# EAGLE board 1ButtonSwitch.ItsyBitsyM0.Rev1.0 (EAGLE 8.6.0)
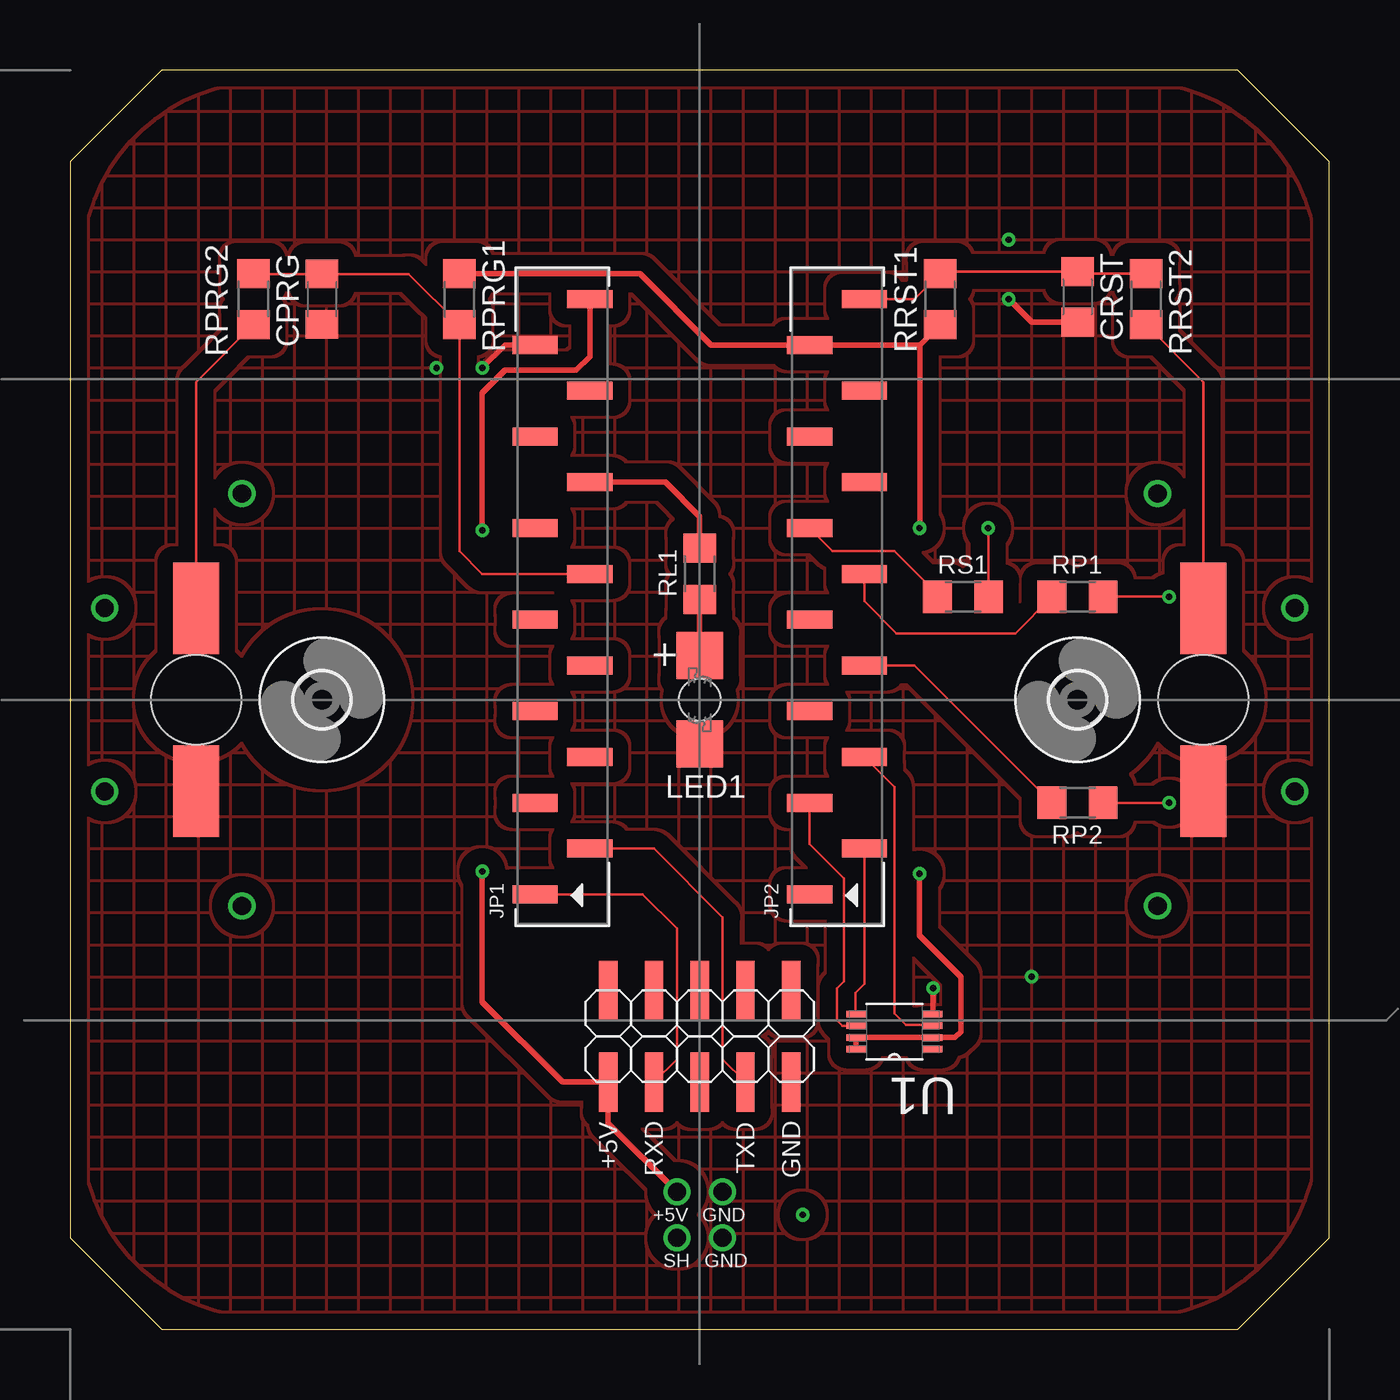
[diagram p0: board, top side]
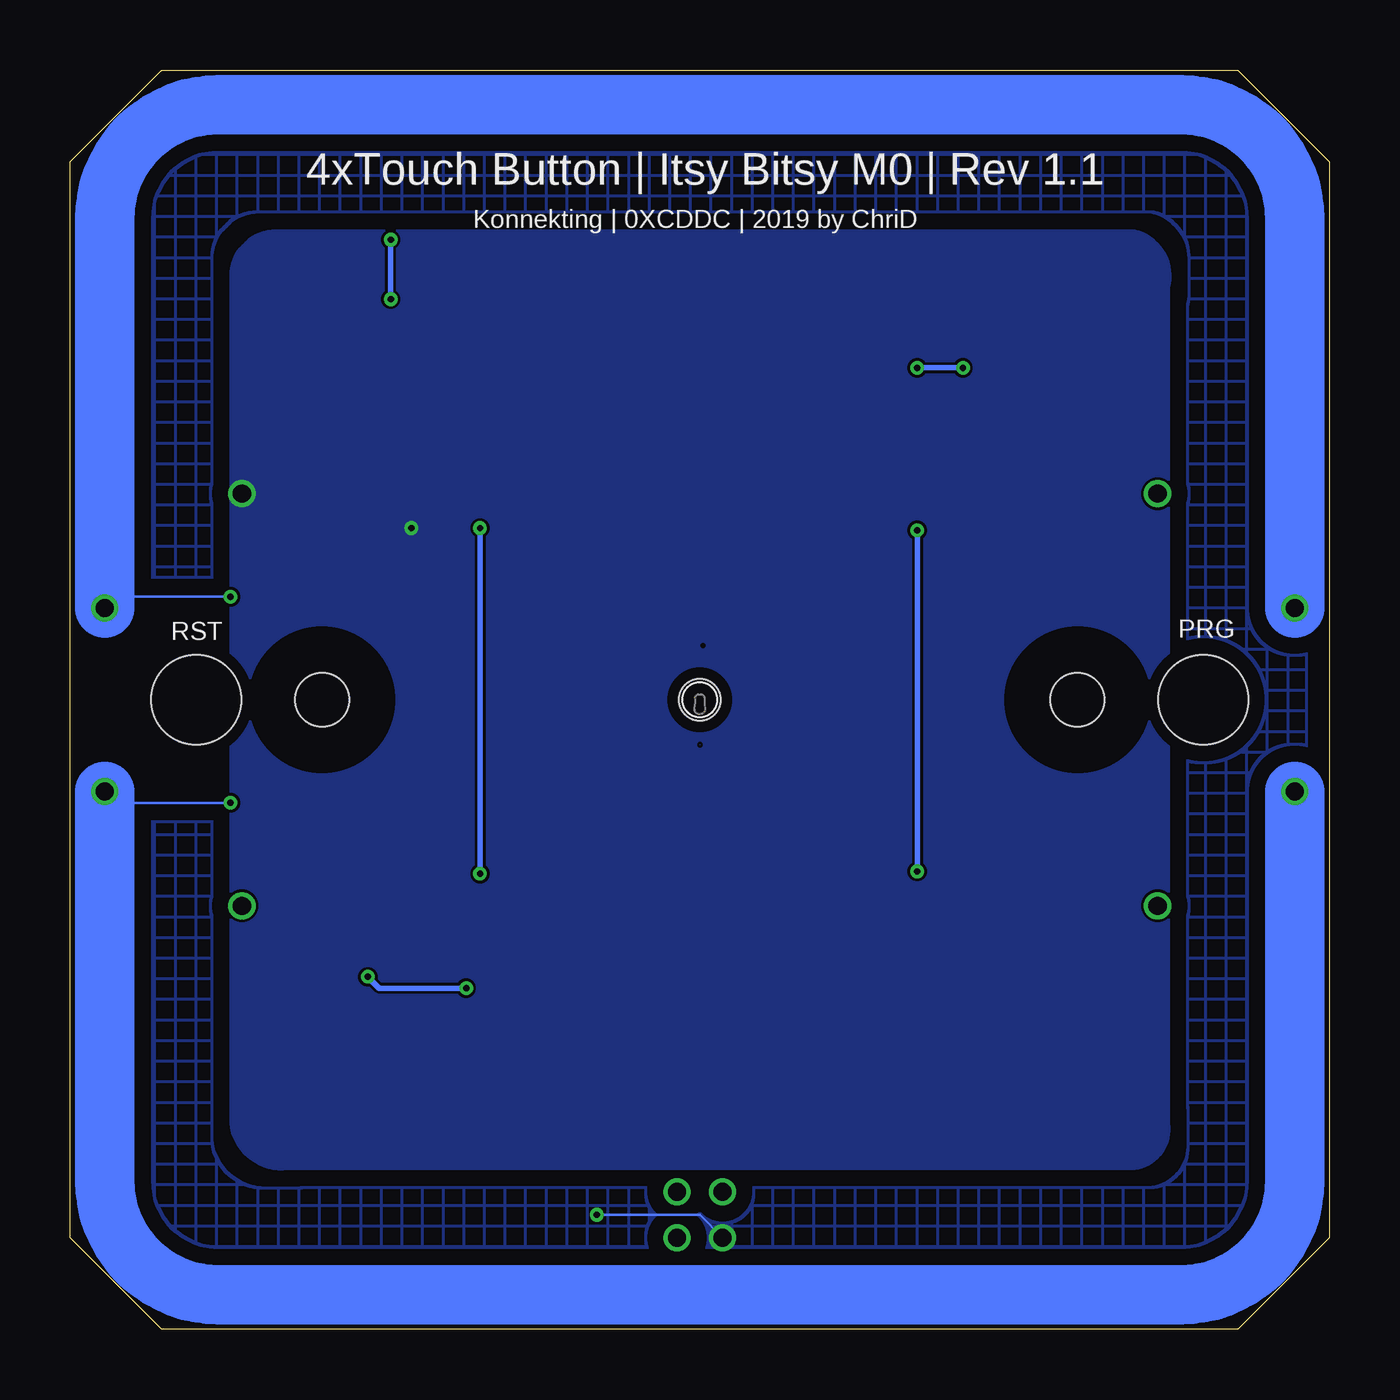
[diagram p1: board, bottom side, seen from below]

Size 69.85 x 69.85 mm. Coordinates in mm from the lower left corner, seen from the top.
Outline: 5.08,69.85 64.77,69.85 69.85,64.77 69.85,5.08 64.77,0 5.08,0 0,5.08 0,64.77 5.08,69.85
Outline: 6.34,69.84 5.08,69.85
Copper layers (1*16): Top 0.035mm / dielectric 1.5mm / Bottom 0.035mm
Design rules "konnektduino": minimum track width 6mil, minimum drill 0.35mm, track to track 6mil, track to pad 6mil, pad to pad 6mil, via to via 6mil, smd to smd 6mil, copper to edge 25mil, drill to drill 6mil, minimum pad ring 10mil, minimum via ring 8mil, stop-mask expansion 1mil, vias tented up to drill 25mil, thermal gap 10mil
Holes 5 mm at 62.87,34.92 6.99,34.92

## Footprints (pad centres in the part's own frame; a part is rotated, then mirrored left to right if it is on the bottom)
C1206 = smd 1.6 x 1.8: 1 -1.4,0; 2 1.4,0
SMD2,54-5,08 = smd 2.54 x 5.08: 1 0,0
1X14_SMT = smd 1 x 2.5: 1 -16.51,1.52; 2 -13.97,-1.52; 3 -11.43,1.52; 4 -8.89,-1.52; 5 -6.35,1.52; 6 -3.81,-1.52; 7 -1.27,1.52; 8 1.27,-1.52; 9 3.81,1.52; 10 6.35,-1.52; 11 8.89,1.52; 12 11.43,-1.52; 13 13.97,1.52; 14 16.51,-1.52
P47F-BOTTOM = smd 2.6 x 2.6: A -2.45,0; C 2.45,0 | hole 2.3: 0,0
R1206 = smd 1.6 x 1.803: 1 -1.422,0; 2 1.422,0
2X05SMD = smd 1.016 x 3.302: 1 -1.27,-3.81; 2 -1.27,1.27; 3 1.27,-3.81; 4 1.27,1.27; 5 3.81,-3.81; 6 3.81,1.27; 7 6.35,-3.81; 8 6.35,1.27; 9 8.89,-3.81; 10 8.89,1.27
SOP65P490X110-8N = smd 1.067 x 0.356: 1 -2.134,0.965; 2 -2.134,0.33; 3 -2.134,-0.33; 4 -2.134,-0.965; 5 2.134,-0.965; 6 2.134,-0.33; 7 2.134,0.33; 8 2.134,0.965
3,0 = hole 3: 0,0

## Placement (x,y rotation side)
CPRG  100nF  [C1206]  13.97,57.15 270 top
CRST  100nF  [C1206]  55.88,57.28 270 top
GND_NRST  0  [SMD2,54-5,08]  6.99,29.84 0 top
GND_PRG  0  [SMD2,54-5,08]  62.87,29.84 0 top
JP1  [1X14_SMT]  27.3,40.64 90 top
JP2  [1X14_SMT]  42.55,40.64 90 top
LED1  LWP4-BOTTOM  [P47F-BOTTOM]  34.92,34.92 270 top
PAD_NRST  0  [SMD2,54-5,08]  62.87,40.01 0 top
PAD_PRG  0  [SMD2,54-5,08]  6.99,40.01 0 top
RL1  330E  [R1206]  34.92,41.91 270 top
RP1  1k  [R1206]  55.88,40.64 180 top
RP2  1k  [R1206]  55.88,29.21 180 top
RPRG1  10k  [R1206]  21.59,57.15 90 top
RPRG2  330E  [R1206]  10.16,57.15 270 top
RRST1  10k  [R1206]  48.26,57.15 270 top
RRST2  330E  [R1206]  59.69,57.15 270 top
RS1  1k  [R1206]  49.53,40.64 180 top
SAM12235-ND  SIEMENS BCU  [2X05SMD]  31.11,17.53 0 top
U1  MAX31723MUA+T  [SOP65P490X110-8N]  45.72,16.51 180 top
U$1  [3,0]  13.97,34.92 0 top
U$2  [3,0]  55.88,34.92 0 top

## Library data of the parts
CPRG CRST = rcl; SPICEPREFIX: C
GND_NRST GND_PRG PAD_NRST PAD_PRG = wirepad
JP1 JP2 = pinhead+
LED1 = led
RL1 RP1 RP2 RPRG1 RPRG2 RRST1 RRST2 RS1 = resistor
SAM12235-ND = pinhead
U1 = MAX31723MUA_T (1); AVAILABILITY: Unavailable; DESCRIPTION: Thermostat Â±2Â°C Digital SMD 8-Pin uMAX T/R; MF: Maxim Integrated; MP: MAX31723MUA+T; PACKAGE: MSOP-8 Maxim Integrated; PRICE: None
U$1 U$2 = holes

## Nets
+3V3: JP2.13 RPRG1.2 RRST1.2 U1.2 U1.7 U1.8
+5V: JP1.14 SAM12235-ND.1
A0: JP2.10
A1: JP2.9 RS1.2
A2: JP2.8 RP1.2
A3: JP2.7
A4: JP2.6 RP2.2
A5: JP2.5
D7: JP1.6
D9: JP1.7
D10: CPRG.1 JP1.8 RPRG1.1 RPRG2.1
D11: JP1.9
D12: JP1.10 RL1.1
D13: JP1.11
GND: CPRG.2 CRST.2 GND_NRST.1 GND_PRG.1 JP1.13 LED1.C SAM12235-ND.9 U1.4
MISO: JP2.2 U1.5
MOSI: JP2.3 U1.6
N$19: LED1.A RL1.2
PRG: PAD_PRG.1 RPRG2.2
RESET: PAD_NRST.1 RRST2.2
RST: CRST.1 JP2.14 RRST1.1 RRST2.1
SCK: JP2.4 U1.3
SCL: JP1.4
SDA: JP1.3
SENS_1: RS1.1
SENS_PROX_1: RP1.1
SENS_PROX_2: RP2.1
USART1_RX: JP1.1 SAM12235-ND.3
USART1_TX: JP1.2 SAM12235-ND.7

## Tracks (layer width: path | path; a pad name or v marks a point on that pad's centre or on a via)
+3V3  (via drill 0.35)
  Top 0.305: 47.14,54.61 JP2.13 35.56,54.61 31.6,58.57 RPRG1.2 | 47.14,54.61 RRST1.2 | U1.8 U1.7 U1.2 49.07,16.18 49.4,16.51 49.4,19.56 47.12,21.84 v47.12,25.27 | 47.14,54.61 47.14,44.48 v47.12,44.45
  Bottom 0.305: v47.12,44.45 v47.12,25.27
+5V  (via drill 0.35, 1)
  Top 0.305: JP1.14 28.82,53.97 28.07,53.21 24.13,53.21 22.86,51.94 v22.86,44.32 | v22.86,25.4 22.86,18.16 27.3,13.72 SAM12235-ND.1 29.84,11.43 v33.66,7.62
  Bottom 0.305: v22.86,44.32 v22.86,25.4
A1
  Top 0.152: JP2.9 42.3,43.18 45.72,43.18 48.11,40.79 RS1.2
A2
  Top 0.152: JP2.8 44.06,40.39 45.85,38.61 52.43,38.61 RP1.2
A4
  Top 0.152: JP2.6 46.84,36.83 RP2.2
D10
  Top 0.152: RPRG2.1 10.18,58.55 CPRG.1 18.77,58.55 RPRG1.1 21.59,43.18 22.86,41.91 JP1.8
D12
  Top 0.305: RL1.1 34.92,45.09 33.02,46.99 JP1.10
GND  (via drill 0.35, 1)
  Top 0.305: JP1.13 24.13,54.61 v22.86,53.34 | CRST.2 53.34,55.88 v52.07,57.15 | U1.4 47.85,18.9 v47.88,18.92
  Bottom 0.305: v22.86,53.34 v20.32,53.34 | v52.07,57.15 v52.07,60.45 | v47.88,18.92 52.7,18.92 v53.34,19.56
  other vias: 36.2,7.62 36.2,5.08
  pour Top (isolate 0.889, rank 6, no thermals, hatched): 0.64,10.79 arc90 10.79,0.64 59.05,0.64 arc90 69.22,10.79 69.22,59.05 arc90 59.05,69.22 10.79,69.22 arc90 0.64,59.05
MISO
  Top 0.152: JP2.2 44.06,19.17 43.56,18.67 43.56,17.5 U1.5
MOSI
  Top 0.152: JP2.3 41.02,26.92 42.93,25.02 42.93,19.3 42.55,18.92 42.55,17.14 42.85,16.84 U1.6
N$19
  Top 0.305: RL1.2 LED1.A
PRG
  Top 0.152: PAD_PRG.1 6.99,52.55 RPRG2.2
RESET
  Top 0.152: PAD_NRST.1 62.87,52.55 RRST2.2
RST
  Top 0.152: RRST2.1 55.99,58.57 CRST.1 48.37,58.68 RRST1.1 46.84,57.15 JP2.14
SCK
  Top 0.152: JP2.4 45.72,30.09 45.72,17.53 46.35,16.89 47.8,16.89 U1.3
SENS_1  (via drill 0.35, 1)
  Top 0.152: RS1.1 50.95,44.42 v50.93,44.45
  other vias: 60.33,46.35
  pour Bottom: 8.89,57.78 8.89,11.43 arc90 10.79,8.89 57.78,8.89 arc90 60.96,11.43 60.96,58.42 arc90 58.42,60.96 10.79,60.96 arc90
SENS_2  (via drill 1)
  other vias: 9.53,46.35
SENS_3  (via drill 1)
  other vias: 60.33,23.5
SENS_4  (via drill 1)
  other vias: 9.53,23.5
SENS_PROX_1  (via drill 0.35, 1)
  Top 0.152: RP1.1 v60.96,40.64
  Bottom 0.152: v60.96,40.64 67.31,40.64 v67.94,40.01
  Bottom 3.302: v1.91,40.01 1.91,61.59 arc-90 8.26,67.94 61.59,67.94 arc-90 67.94,61.59 v67.94,40.01
SENS_PROX_2  (via drill 0.35, 1)
  Top 0.152: RP2.1 v60.96,29.21
  Bottom 0.152: v60.96,29.21 67.31,29.21 v67.94,29.84
  Bottom 3.302: v1.91,29.84 1.91,8.26 arc90 8.26,1.91 61.59,1.91 arc90 67.94,8.26 v67.94,29.84
SHIELD_OR_GND  (via drill 0.35, 1)
  Bottom 0.152: v33.66,5.08 34.92,6.35 v40.64,6.35
  pour Bottom (isolate 0.889, rank 6, no thermals, hatched): 1.27,6.99 arc90 6.99,1.27 61.59,2.54 arc90 67.31,8.26 67.31,61.59 arc90 61.59,67.31 6.99,67.31 arc90 1.27,61.59
USART1_RX
  Top 0.152: JP1.1 31.75,24.13 33.66,22.23 33.66,14.99 SAM12235-ND.3
USART1_TX
  Top 0.152: SAM12235-ND.7 36.2,14.99 36.2,22.86 32.38,26.67 JP1.2

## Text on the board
tNames: + | +5V | RXD | TXD | GND | +5V | GND | SH | GND
bNames: 4xTouch Button | Itsy Bitsy M0 | Rev 1.1 | Konnekting | 0XCDDC | 2019 by ChriD | PRG | RST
